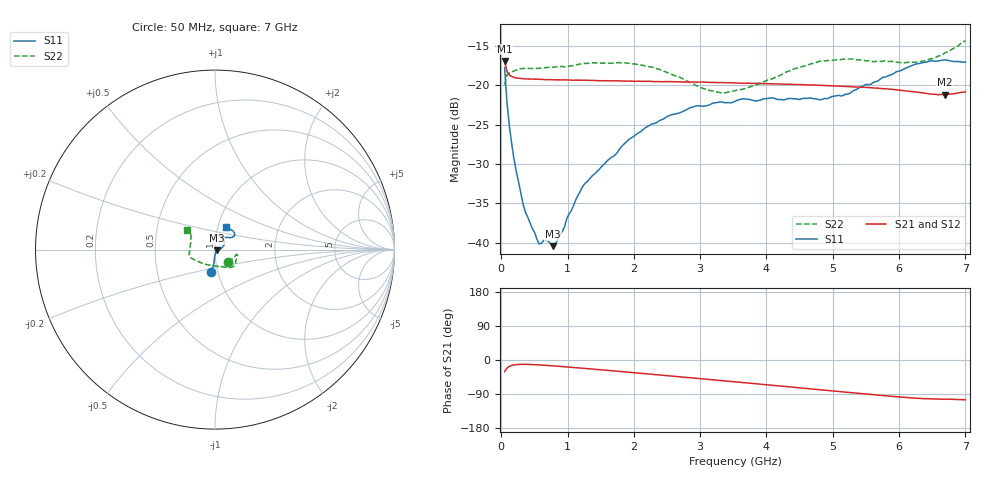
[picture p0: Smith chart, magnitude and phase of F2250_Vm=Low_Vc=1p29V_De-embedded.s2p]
! Integrated Device Technology
! Corporate Headquarters
! 6024 Silver Creek Valley Road
! San Jose, CA 95138  USA
! Phone:  1-408-284-8200
! Toll Free:  1-800-223-1366
! Webpage:  http://www.idt.com/
! Timing and RF Division
! 515 Groton Road, Suite 102
! Westford, MA 01886-6024
! Device:  F2250
! Description: Voltage Variable RF Attenuator
! Frequency:  50.0 -  6000.00 MHz
! Package:  3x3 mm Thin QFN Plastic Package: 16 pin
! Ports:  2 RF, 3 DC
!  Pin  1  = GND
!  Pin  2  = NC
!  Pin  3  = RF1  = Port 1
!  Pin  4  = NC
!  Pin  5  = GND
!  Pin  6  = GND
!  Pin  7  = GND
!  Pin  8  = GND
!  Pin  9  = NC
!  Pin 10  = RF2  = Port 2
!  Pin 11  = NC
!  Pin 12  = GND
!  Pin 13  = GND
!  Pin 14  = VCNTRL
!  Pin 15  = VDD
!  Pin 16  = VMODE
! Vcntrl:  1.290 Volts
! Vmode:  +0.000 Volts
! Vdd:  +3.30  Volts
! Current:  1.196 mA
! Data:  The device was measured on a the F2250 evaluation board which has
!  individual transmission lines to the RF pins.  Data was collected
!  using a calibrated network analyzer.  The evaluation board was
!  de-embedded using a TRL calibration technique.
!  The reference plane is the edge of the package pin.
! Misc:  SN 10
!  Action Tracker AT0258
! Date Measured:  2014-11-26
! Date:  2015-10-15  MJV
! Note:
!  Integrated Device Technology supplies this data as a sample of measured
!  data at the package pin for this product.  Your particular data for this
!  product may vary.
!  Data was taken at 25 degrees C.
!  Integrated Device Technology reserves the right to change this data at anytime.
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# GHz S dB R 50
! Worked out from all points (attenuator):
!   201 points, 50 MHz to 7 GHz, reference 50 ohm
!   highest |S21| = -16.91 dB at 50 MHz (marker M1); lowest = -21.2 dB at 6.687 GHz (marker M2)
!   lowest |S11| = -40.4 dB at 779.8 MHz (marker M3), VSWR 1.02, Z = 50.9 - j0.43 ohm
!   |S11| at or under -10 dB: start of sweep to end of sweep
!   |S22| runs from -21.0 to -14.3 dB; largest |S21 - S12| = 0.00035
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0.05  -17.76 -100.3  -16.91 -30.3  -16.91 -30.3  -19.94 -43.1
0.08475  -22.07 -94.3  -18.23 -21.5  -18.22 -21.5  -18.69 -21.1
0.15425  -27.29 -93.8  -18.87 -14.5  -18.87 -14.5  -18.34 -13.2
0.22375  -30.84 -88.2  -19.07 -12.2  -19.08 -12.2  -18.10 -12.6
0.328  -35.08 -78.9  -19.16 -11.4  -19.18 -11.4  -17.87 -12.8
0.57125  -40.17 -50.3  -19.24 -13.0  -19.25 -13.0  -17.86 -17.7
0.6755  -39.68 -42.1  -19.30 -14.2  -19.28 -14.2  -17.76 -20.2
0.77975  -40.44 -26.4  -19.31 -15.5  -19.30 -15.5  -17.72 -22.9
0.91875  -38.59 -15.3  -19.33 -17.3  -19.33 -17.3  -17.60 -26.8
0.98825  -36.95 -18.9  -19.33 -18.3  -19.33 -18.3  -17.62 -28.1
1.2315  -32.80 -3.0  -19.36 -21.8  -19.36 -21.8  -17.25 -33.2
1.9265  -26.88 19.0  -19.47 -32.3  -19.46 -32.3  -17.23 -44.0
2.37825  -24.53 30.1  -19.53 -39.3  -19.54 -39.3  -17.96 -52.0
2.86475  -22.82 44.8  -19.60 -47.1  -19.60 -47.1  -19.71 -67.8
3.14275  -22.49 52.6  -19.64 -51.5  -19.64 -51.5  -20.66 -83.3
3.525  -22.04 63.8  -19.72 -57.7  -19.71 -57.7  -20.69 -109.4
4.7065  -21.71 68.1  -19.96 -76.9  -19.98 -76.9  -17.23 -159.0
5.15825  -21.30 52.8  -20.14 -84.3  -20.15 -84.3  -16.69 -167.6
5.85325  -18.74 36.0  -20.49 -95.3  -20.49 -95.3  -16.99 178.4
6.33975  -17.17 38.0  -20.96 -101.6  -20.94 -101.8  -16.97 160.9
6.68725  -16.78 46.7  -21.21 -103.3  -21.21 -103.3  -15.92 147.9
7  -17.07 62.8  -20.83 -105.0  -20.84 -105.0  -14.31 144.7
